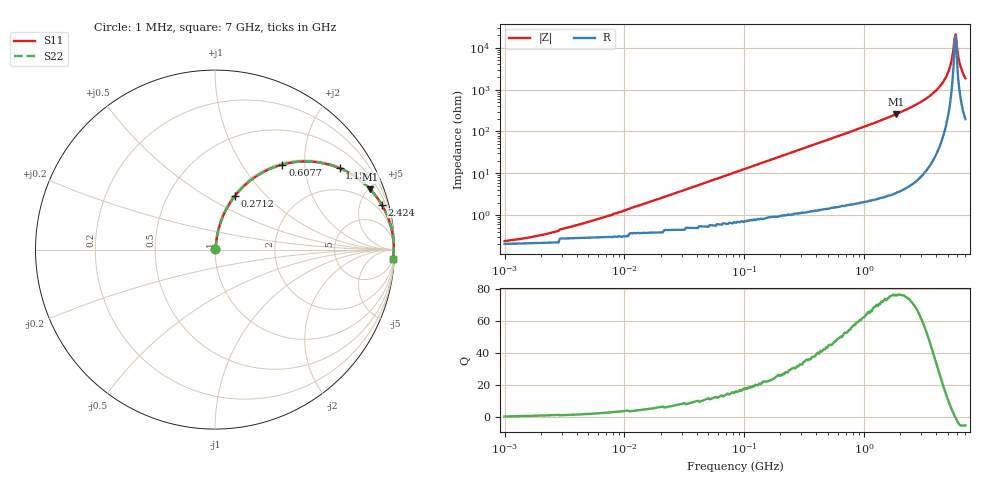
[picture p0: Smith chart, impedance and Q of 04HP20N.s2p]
# MHz S MA R 50
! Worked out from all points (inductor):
!   385 points, 1 MHz to 7 GHz, reference 50 ohm
!   read as one part in series: L = 20 nH near 7.263 MHz
!   highest Q = 76.4 at 1.838 GHz (marker M1), where L = 22.3 nH
!   self-resonance near 5.688 GHz
!   S11 on the Smith chart (normalised r, x): 1 MHz: 1.00, +0.00; 271.2 MHz: 1.02, +0.68; 607.7 MHz: 1.03, +1.54; 1.159 GHz: 1.05, +3.03; 2.424 GHz: 1.10, +7.39; 7 GHz: 5, -37
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1  0.002453 30.7  0.998 -0.1  0.998 -0.1  0.002453 30.7
4.374  0.006119 63.3  0.997 -0.3  0.997 -0.3  0.006119 63.3
19.575  0.025 79.3  0.996 -1.4  0.996 -1.4  0.025 79.3
85.617  0.106 80.3  0.988 -6.1  0.988 -6.1  0.106 80.3
271.16  0.32 69.5  0.937 -18.7  0.937 -18.7  0.32 69.5
365.931  0.415 63.9  0.899 -24.5  0.899 -24.5  0.415 63.9
607.702  0.605 51.6  0.784 -37.2  0.784 -37.2  0.605 51.6
1158.944  0.829 33.1  0.546 -56.0  0.546 -56.0  0.829 33.1
1637.803  0.909 23.9  0.406 -65.3  0.406 -65.3  0.909 23.9
1837.926  0.928 21.2  0.361 -68.1  0.361 -68.1  0.928 21.2
2423.747  0.962 15.1  0.26 -74.1  0.26 -74.1  0.962 15.1
3586.848  0.988 7.7  0.135 -81.0  0.135 -81.0  0.988 7.7
4622.31  0.995 3.5  0.062 -83.4  0.062 -83.4  0.995 3.5
5187.11  0.996 1.7  0.03 -81.2  0.03 -81.2  0.996 1.7
5431.903  0.996 1.0  0.017 -76.0  0.017 -76.0  0.996 1.0
5558.598  0.996 0.6  0.011 -68.4  0.011 -68.4  0.996 0.6
5688.248  0.996 0.2  0.005852 -44.8  0.005852 -44.8  0.996 0.2
5820.923  0.996 -0.1  0.004785 27.0  0.004785 27.0  0.996 -0.1
6095.627  0.995 -0.8  0.016 72.1  0.016 72.1  0.995 -0.8
6237.803  0.995 -1.2  0.022 76.3  0.022 76.3  0.995 -1.2
6684.539  0.994 -2.3  0.041 80.3  0.041 80.3  0.994 -2.3
7000  0.993 -3.0  0.053 80.9  0.053 80.9  0.993 -3.0
